(* Logix 5000 AddOnInstructionDefinition export Banner_WLS_PD_v4; software revision 33.00 *)

TYPE Banner_WLS_CC_v4 :   // Tags to control color for a WLS Pro
STRUCT
   Animation : SINT;   // 0 = Off, 1 = Steady, 2 = Flash, 3 = 2 Color Flash, 4 = 2 Color Shift, 5 = Ends Steady, 6 = Ends Flash, 7 = Scroll, 8 = Center Bounce, 9 = Bounce, 10 = Center Bounce, 11 = Intensity Sweep, 12 = 2 Color Sweep, 13 = Spectrum. WLS15 Only 14 = Level Steady, 15 = Level Flash.
   Color_1 : SINT;   // 0 = Green, 1 = Red, 2 = Orange, 3 = Amber, 4 = Yellow, 5 = Lime Green, 6 = Spring Green, 7 = Cyan, 8 = Sky Blue, 9 = Blue, 10 = Violet, 11 = Magneta, 12 = Rose, 13 = Daylight White, 14 = Custom 1, 15 = Custom 2, 16 = Incandescent, 17 = Warm White, 18 = Flourescent, 19 = Neutral White, 20 = Cool White.
   Color_1_Intensity : SINT;   // 0 = High, 1 = Low, 2 = Medium, 3 = Off, 4 = Custom.
   Speed : SINT;   // 0 = Medium, 1 = Fast, 2 = Slow, 3 = Custom.
   Pulse_Pattern : SINT;   // 0 = Normal, 1 = Strobe, 2 = Three Pulse, 3 = SOS, 4 = Random.
   Color_2 : SINT;   // 0 = Green, 1 = Red, 2 = Orange, 3 = Amber, 4 = Yellow, 5 = Lime Green, 6 = Spring Green, 7 = Cyan, 8 = Sky Blue, 9 = Blue, 10 = Violet, 11 = Magneta, 12 = Rose, 13 = Daylight White, 14 = Custom 1, 15 = Custom 2, 16 = Incandescent, 17 = Warm White, 18 = Flourescent, 19 = Neutral White, 20 = Cool White.
   Color_2_Intensity : SINT;   // 0 = High, 1 = Low, 2 = Medium, 3 = Off, 4 = Custom.
   ScrollBounce : SINT;   // 0 = Solid, 1 = Blended Tail, 2 = Center Blended.
   Percent_Width_C1 : SINT;   // 1 to 100% of Color 1.
   Direction : SINT;   // 0 = Forward, 1 = Backward.
END_STRUCT
END_TYPE

TYPE Banner_WLS_PDIO_v4 :   // Process data for a Banner WLS Pro unit. This includes four process data types.
STRUCT
   Segment_Mode : SINT[11];   // 0 = Off, 1 = On, 2 = Flash, 3 = Animation.
   Run_Mode : Banner_WLS_CC_v4;   // Tags for Run Mode control
   Level_Mode : INT;   // Value describing level of the device range. See Level Mode Parameter for more information.
   Dim_Blend_Mode : INT;   // Value describing the amount of blend between colors selected in Dim and Blend Mode parameter data.
   Gauge_Mode_Value : INT;   // Value describing the position of the main animation.
   LED_Mode : SINT[65];   // 0 = Off, 1 = Green, 2 = Red, 3 = Orange, 4 = Amber, 5 = Yellow, 6 = Lime Green, 7 = Spring Green, 8 = Cyan, 9 = Sky Blue, 10 = Blue, 11 = Violet, 12 = Magneta, 13 = Rose, 14 = Daylight White, 15 = Custom 1.
   Transfer_Data : SINT[32];   // Data array to send the correct state of the process data output to the IO-Link master.
END_STRUCT
END_TYPE

ADD_ON_INSTRUCTION Banner_WLS_PD_v4   (* revision 4.0, vendor Banner Engineering *)
// Takes the raw SINT information and converts that data into actual information.
VAR_IN_OUT
   PROCESS_DATA : Banner_WLS_PDIO_v4; {required}
END_VAR
VAR_INPUT
   Byte_Swap : BOOL; {required}   // Swap the LSB and the MSB with each other.
   Operation_Mode : INT; {required}   // 0= Segment, 1 = Run, 2 = Level, 3 = Variable Color, 4 = Position, 5 = LED
END_VAR
VAR
   Data_Byte : SINT[64]; {access None}
   Temp_Data : SINT[64]; {access None}
   Index2 : DINT := 31; {access None}
   Index1 : DINT; {access None}
END_VAR

ROUTINE Logic   (* ladder *)
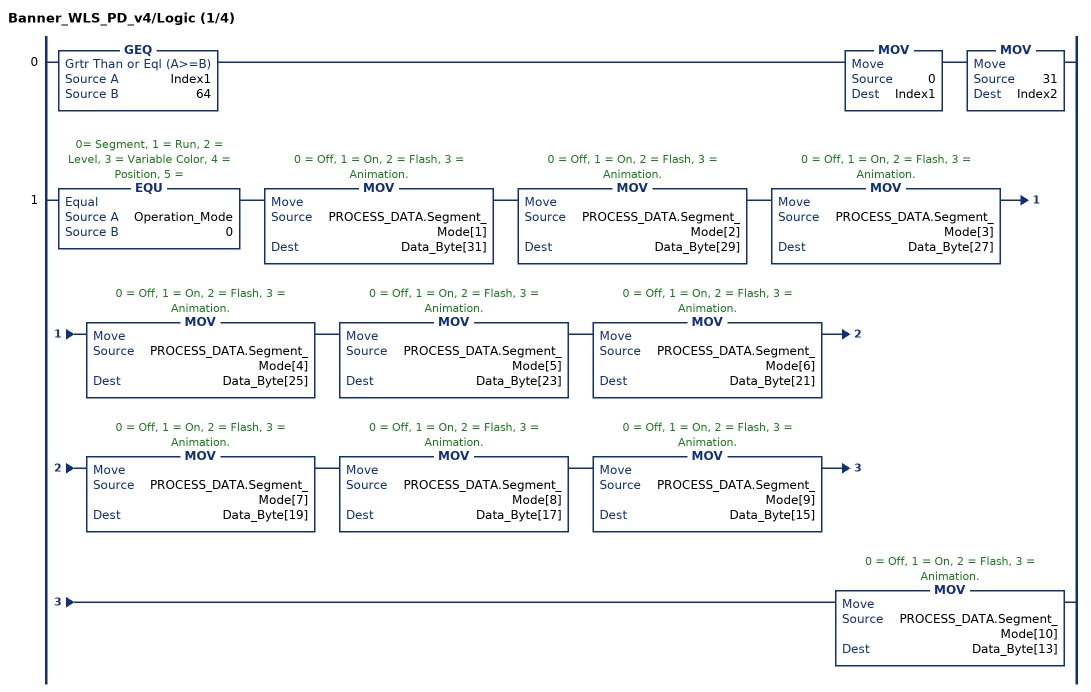
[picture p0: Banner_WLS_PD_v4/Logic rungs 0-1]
   0: GEQ(Index1,64)MOV(0,Index1)MOV(31,Index2);
   1: EQU(Operation_Mode,0)MOV(PROCESS_DATA.Segment_Mode[1],Data_Byte[31])MOV(PROCESS_DATA.Segment_Mode[2],Data_Byte[29])MOV(PROCESS_DATA.Segment_Mode[3],Data_Byte[27])MOV(PROCESS_DATA.Segment_Mode[4],Data_Byte[25])MOV(PROCESS_DATA.Segment_Mode[5],Data_Byte[23])MOV(PROCESS_DATA.Segment_Mode[6],Data_Byte[21])MOV(PROCESS_DATA.Segment_Mode[7],Data_Byte[19])MOV(PROCESS_DATA.Segment_Mode[8],Data_Byte[17])MOV(PROCESS_DATA.Segment_Mode[9],Data_Byte[15])MOV(PROCESS_DATA.Segment_Mode[10],Data_Byte[13]);
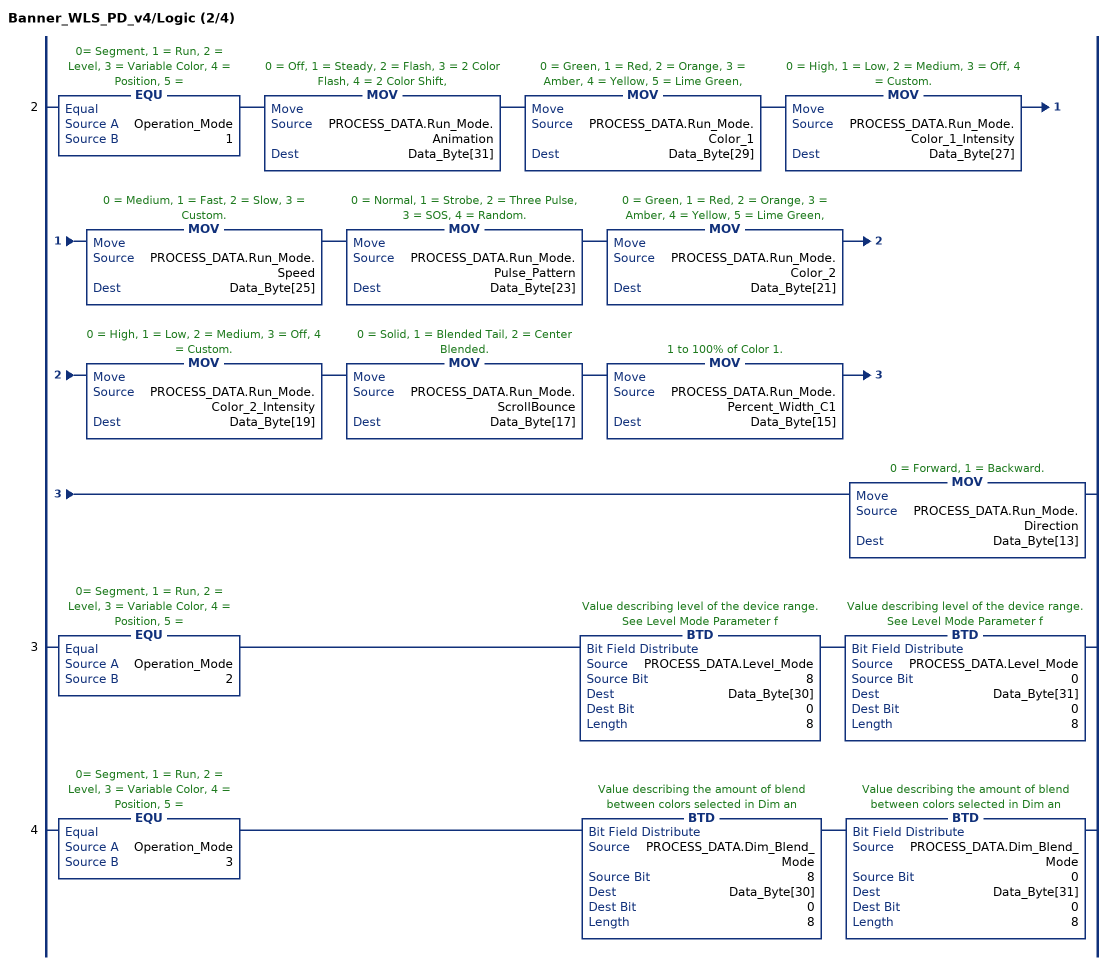
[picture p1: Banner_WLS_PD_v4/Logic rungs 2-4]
   2: EQU(Operation_Mode,1)MOV(PROCESS_DATA.Run_Mode.Animation,Data_Byte[31])MOV(PROCESS_DATA.Run_Mode.Color_1,Data_Byte[29])MOV(PROCESS_DATA.Run_Mode.Color_1_Intensity,Data_Byte[27])MOV(PROCESS_DATA.Run_Mode.Speed,Data_Byte[25])MOV(PROCESS_DATA.Run_Mode.Pulse_Pattern,Data_Byte[23])MOV(PROCESS_DATA.Run_Mode.Color_2,Data_Byte[21])MOV(PROCESS_DATA.Run_Mode.Color_2_Intensity,Data_Byte[19])MOV(PROCESS_DATA.Run_Mode.ScrollBounce,Data_Byte[17])MOV(PROCESS_DATA.Run_Mode.Percent_Width_C1,Data_Byte[15])MOV(PROCESS_DATA.Run_Mode.Direction,Data_Byte[13]);
   3: EQU(Operation_Mode,2)BTD(PROCESS_DATA.Level_Mode,8,Data_Byte[30],0,8)BTD(PROCESS_DATA.Level_Mode,0,Data_Byte[31],0,8);
   4: EQU(Operation_Mode,3)BTD(PROCESS_DATA.Dim_Blend_Mode,8,Data_Byte[30],0,8)BTD(PROCESS_DATA.Dim_Blend_Mode,0,Data_Byte[31],0,8);
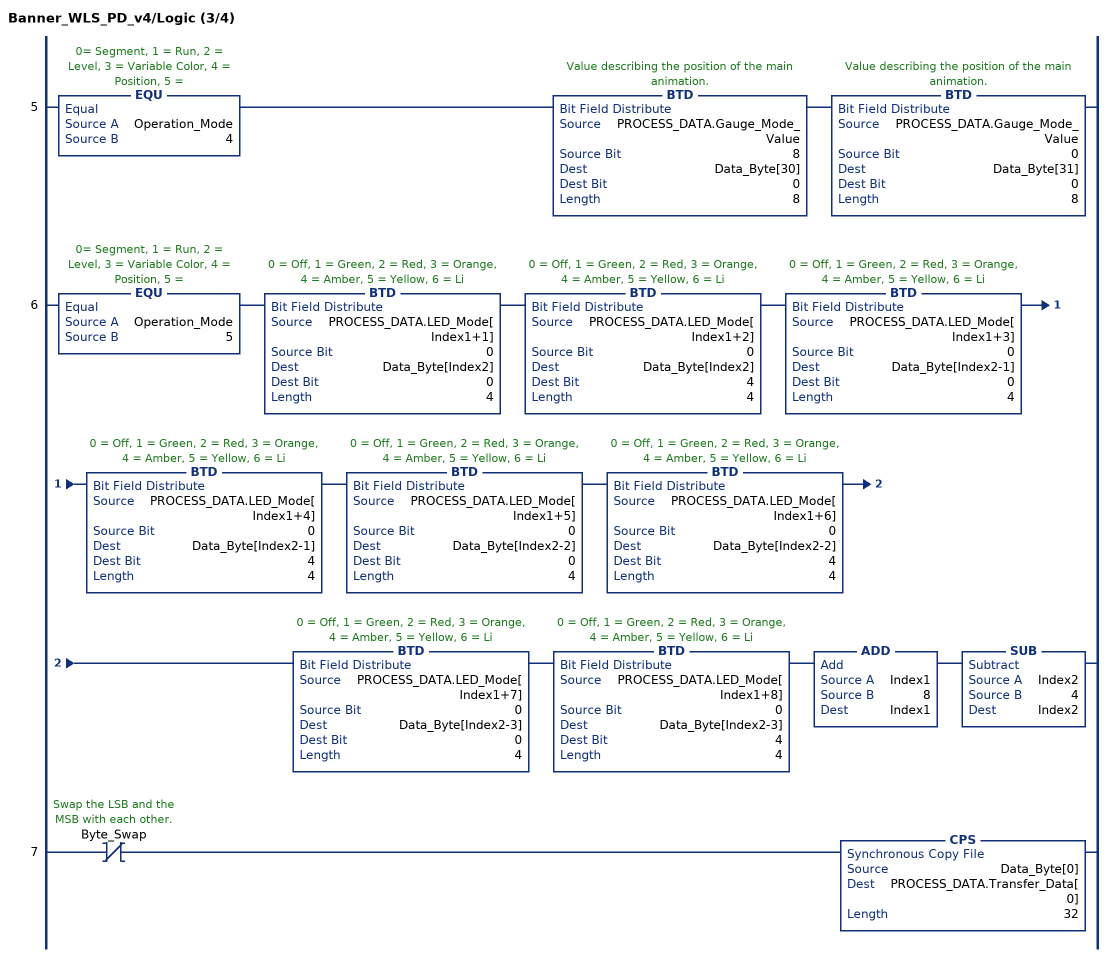
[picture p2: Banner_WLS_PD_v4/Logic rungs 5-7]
   5: EQU(Operation_Mode,4)BTD(PROCESS_DATA.Gauge_Mode_Value,8,Data_Byte[30],0,8)BTD(PROCESS_DATA.Gauge_Mode_Value,0,Data_Byte[31],0,8);
   6: EQU(Operation_Mode,5)BTD(PROCESS_DATA.LED_Mode[Index1+1],0,Data_Byte[Index2],0,4)BTD(PROCESS_DATA.LED_Mode[Index1+2],0,Data_Byte[Index2],4,4)BTD(PROCESS_DATA.LED_Mode[Index1+3],0,Data_Byte[Index2-1],0,4)BTD(PROCESS_DATA.LED_Mode[Index1+4],0,Data_Byte[Index2-1],4,4)BTD(PROCESS_DATA.LED_Mode[Index1+5],0,Data_Byte[Index2-2],0,4)BTD(PROCESS_DATA.LED_Mode[Index1+6],0,Data_Byte[Index2-2],4,4)BTD(PROCESS_DATA.LED_Mode[Index1+7],0,Data_Byte[Index2-3],0,4)BTD(PROCESS_DATA.LED_Mode[Index1+8],0,Data_Byte[Index2-3],4,4)ADD(Index1,8,Index1)SUB(Index2,4,Index2);
   7: XIO(Byte_Swap)CPS(Data_Byte[0],PROCESS_DATA.Transfer_Data[0],32);
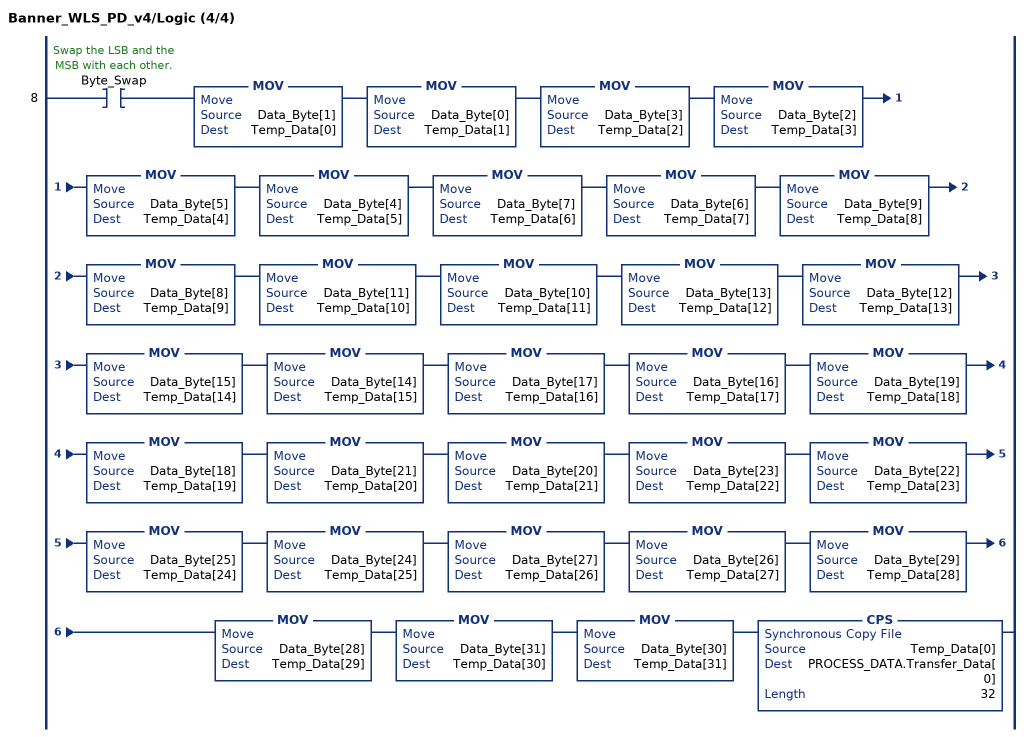
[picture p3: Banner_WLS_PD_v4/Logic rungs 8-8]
   8: XIC(Byte_Swap)MOV(Data_Byte[1],Temp_Data[0])MOV(Data_Byte[0],Temp_Data[1])MOV(Data_Byte[3],Temp_Data[2])MOV(Data_Byte[2],Temp_Data[3])MOV(Data_Byte[5],Temp_Data[4])MOV(Data_Byte[4],Temp_Data[5])MOV(Data_Byte[7],Temp_Data[6])MOV(Data_Byte[6],Temp_Data[7])MOV(Data_Byte[9],Temp_Data[8])MOV(Data_Byte[8],Temp_Data[9])MOV(Data_Byte[11],Temp_Data[10])MOV(Data_Byte[10],Temp_Data[11])MOV(Data_Byte[13],Temp_Data[12])MOV(Data_Byte[12],Temp_Data[13])MOV(Data_Byte[15],Temp_Data[14])MOV(Data_Byte[14],Temp_Data[15])MOV(Data_Byte[17],Temp_Data[16])MOV(Data_Byte[16],Temp_Data[17])MOV(Data_Byte[19],Temp_Data[18])MOV(Data_Byte[18],Temp_Data[19])MOV(Data_Byte[21],Temp_Data[20])MOV(Data_Byte[20],Temp_Data[21])MOV(Data_Byte[23],Temp_Data[22])MOV(Data_Byte[22],Temp_Data[23])MOV(Data_Byte[25],Temp_Data[24])MOV(Data_Byte[24],Temp_Data[25])MOV(Data_Byte[27],Temp_Data[26])MOV(Data_Byte[26],Temp_Data[27])MOV(Data_Byte[29],Temp_Data[28])MOV(Data_Byte[28],Temp_Data[29])MOV(Data_Byte[31],Temp_Data[30])MOV(Data_Byte[30],Temp_Data[31])CPS(Temp_Data[0],PROCESS_DATA.Transfer_Data[0],32);
END_ROUTINE
END_ADD_ON_INSTRUCTION
